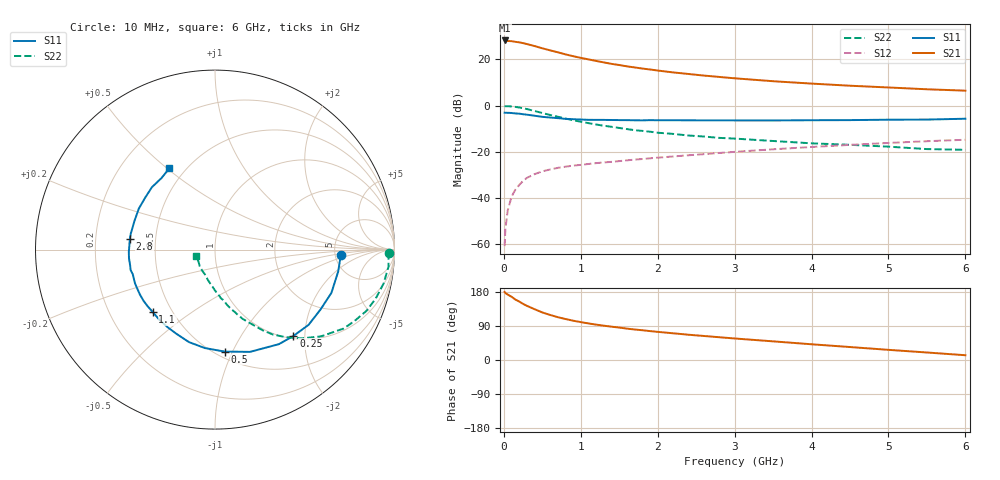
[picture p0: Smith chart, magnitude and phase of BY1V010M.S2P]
! SIEMENS Small Signal Semiconductors
! BFY420
! Si NPN RF SIEGET Grounded Emitter Transistor in MICRO-X
! VCE = 1 V  IC = 10 mA
! Common Emitter S-Parameters:  October  1996
# GHz  S  MA  R  50
!  f  S11  S21  S12  S22
! GHz  MAG  ANG  MAG  ANG  MAG  ANG  MAG  ANG
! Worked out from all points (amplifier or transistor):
!   36 points, 10 MHz to 6 GHz, reference 50 ohm
!   highest |S21| = 28.2 dB at 10 MHz (marker M1)
!   |S21| within 3 dB of that: start of sweep to 459.1 MHz
!   unconditionally stable (mu >= 1): 2.398 GHz to end of sweep
!   at 250 MHz: K = 0.19, MSG = 29.9 dB, |S12| = -32.7 dB
!   at 1.4 GHz: K = 0.77, MSG = 21.2 dB, |S12| = -24.4 dB
!   at 6 GHz: K = 1.11, MAG = 8.6 dB, |S12| = -14.8 dB
!   S11 on the Smith chart (normalised r, x): 10 MHz: 5.62, -0.62; 250 MHz: 1.05, -1.75; 500 MHz: 0.55, -0.93; 1.1 GHz: 0.39, -0.36; 2.8 GHz: 0.35, +0.05; 6 GHz: 0.41, +0.51
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0.01  0.7011 -2.3  25.77 179.4  0.0009 109.1  0.9718 -1.0
0.02  0.6994 -4.3  25.65 176.6  0.0021 91.9  0.9672 -2.0
0.1  0.6919 -20.4  24.89 166.9  0.0106 81.4  0.9581 -11.4
0.15  0.6759 -29.7  24.06 159.5  0.0151 75.9  0.9358 -17.0
0.2  0.669 -38.8  23.47 154.3  0.0191 72.4  0.9097 -22.1
0.25  0.6498 -47.8  22.55 148.1  0.0233 68.2  0.8733 -27.1
0.3  0.6359 -55.9  21.54 142.9  0.0272 65.3  0.8412 -31.5
0.4  0.6024 -71.1  19.49 134.0  0.0327 59.1  0.7633 -39.3
0.5  0.5706 -84.6  17.43 125.5  0.0376 55.2  0.6909 -45.7
0.6  0.5515 -95.9  15.76 119.0  0.0413 52.7  0.6279 -51.0
0.7  0.5354 -105.7  14.31 113.1  0.0447 49.6  0.574 -55.6
0.8  0.5164 -114.4  12.88 108.2  0.0474 47.6  0.5242 -59.3
0.9  0.507 -121.1  11.77 103.8  0.0501 47.0  0.4824 -62.2
1.1  0.4912 -135.0  10.03 96.5  0.0543 45.4  0.4172 -68.1
1.3  0.4898 -144.3  8.62 90.6  0.0587 44.7  0.3658 -72.3
1.6  0.4839 -156.9  7.082 82.8  0.0651 44.1  0.3099 -78.2
2.2  0.4816 -174.3  5.235 70.5  0.079 43.5  0.2436 -87.3
2.8  0.4783 173.1  4.176 60.1  0.094 41.8  0.1998 -95.5
3.5  0.4763 160.3  3.374 49.2  0.113 38.5  0.171 -104.1
4.5  0.4848 143.4  2.696 34.2  0.1409 31.9  0.1413 -117.7
5.5  0.498 126.6  2.257 19.8  0.1692 23.5  0.1142 -143.2
6  0.5193 119.4  2.106 12.6  0.1821 18.9  0.1102 -160.0
